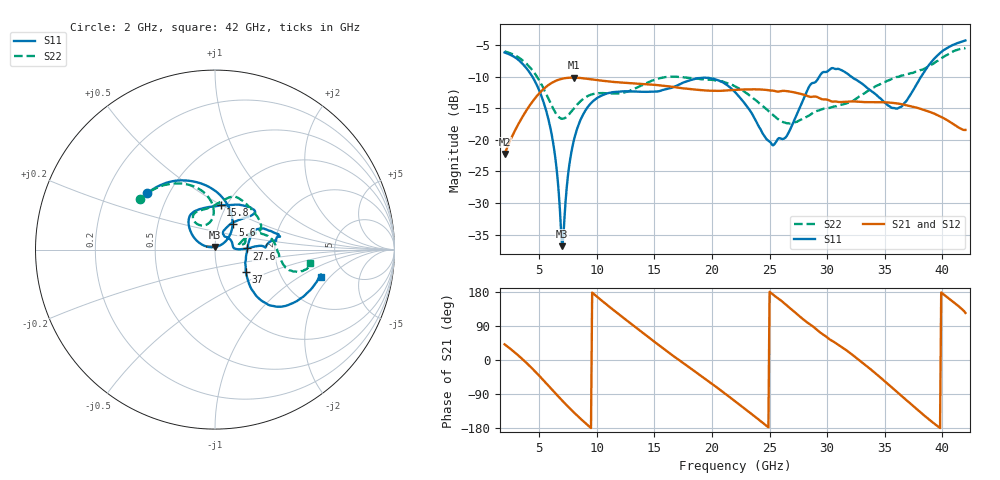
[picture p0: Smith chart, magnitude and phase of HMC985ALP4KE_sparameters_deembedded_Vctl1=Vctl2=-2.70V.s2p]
!s2p File: Measurements: S11, S21, S12, S22
# GHz S dB R 50.0
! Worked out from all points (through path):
!   401 points, 2 GHz to 42 GHz, reference 50 ohm
!   highest |S21| = -10.16 dB at 8 GHz (marker M1); lowest = -22.2 dB at 2 GHz (marker M2)
!   lowest |S11| = -36.8 dB at 7 GHz (marker M3), VSWR 1.03, Z = 49.9 + j1.44 ohm
!   |S11| at or under -10 dB: 4.408 GHz to 29.32 GHz (24.91 GHz wide, 148 % of centre); 32.1 GHz to 38.16 GHz (6.06 GHz wide, 17.3 % of centre)
!   |S22| runs from -17.4 to -5.5 dB; largest |S21 - S12| = 0.00036
!   S11 on the Smith chart (normalised r, x): 2 GHz: 0.38, +0.32; 5.6 GHz: 1.17, +0.34; 15.8 GHz: 0.94, +0.49; 27.6 GHz: 1.43, +0.02; 37 GHz: 1.36, -0.35; 42 GHz: 3.32, -1.59
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2  -6.18 140.2  -22.24 41.3  -22.25 41.3  -6.01 146.1
3.7  -8.25 104.5  -15.92 -2.0  -15.93 -2.0  -7.64 117.4
5.6  -15.34 55.0  -11.62 -61.1  -11.62 -61.1  -12.70 92.2
6.3  -21.52 39.2  -10.79 -84.3  -10.79 -84.3  -15.34 95.4
7  -36.84 91.4  -10.33 -107.1  -10.33 -107.1  -16.68 110.0
8  -20.17 156.2  -10.16 -137.9  -10.16 -137.9  -15.07 125.2
8.7  -16.41 147.1  -10.24 -158.0  -10.24 -158.0  -13.71 125.8
12.2  -12.34 119.6  -10.95 114.0  -10.95 113.9  -12.57 98.5
15.4  -12.31 88.0  -11.37 39.0  -11.37 39.1  -10.28 73.3
15.8  -12.08 82.8  -11.43 29.9  -11.44 29.9  -10.12 71.3
18.4  -10.42 52.1  -12.03 -27.6  -12.03 -27.6  -10.28 53.3
22  -12.44 47.3  -12.11 -108.7  -12.11 -108.7  -11.53 22.4
25.2  -20.74 56.6  -12.21 175.2  -12.21 175.2  -15.94 18.0
26.4  -19.63 5.0  -12.28 146.2  -12.28 146.2  -17.34 12.1
27.6  -15.04 2.0  -12.67 115.4  -12.68 115.4  -16.91 9.4
28.7  -11.02 2.3  -13.19 90.1  -13.20 90.1  -15.81 11.1
31.1  -8.86 13.9  -14.02 37.3  -14.03 37.3  -14.51 22.4
33.3  -11.50 25.6  -14.04 -12.6  -14.04 -12.7  -12.56 22.9
35.4  -14.68 6.3  -14.11 -66.6  -14.11 -66.7  -10.55 15.4
37  -13.52 -35.4  -14.57 -109.1  -14.58 -109.0  -9.58 6.8
39.7  -6.42 -41.9  -16.19 -177.3  -16.19 -177.4  -7.37 -15.5
42  -4.28 -14.2  -18.44 124.3  -18.45 124.3  -5.46 -7.9
